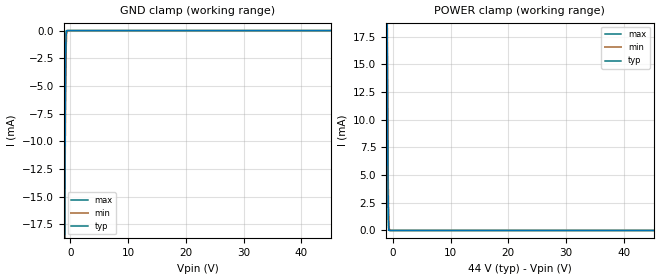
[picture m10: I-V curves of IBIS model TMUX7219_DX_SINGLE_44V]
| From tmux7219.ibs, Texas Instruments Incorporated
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[Model]   TMUX7219_DX_SINGLE_44V
Model_type   Terminator
|   typ   min   max
C_comp   45pF   45pF   45pF
[Voltage Range]   44   39.6   48.4
[Temperature Range]   27   125   -40
[Power Clamp Reference]   44   39.6   48.4
[GND Clamp Reference]   0   0   0
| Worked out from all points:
|   GND clamp passes 1 mA (typ) near -0.77 V on its own axis
|   POWER clamp passes 1 mA (typ) near -0.77 V on its own axis
[GND Clamp]
|   Voltage   I(typ)   I(min)   I(max)
-30V      -4.646A    -4.808A    -4.649A
-1.02V    -22.01mA   -24.41mA   -19.81mA
-930mV    -11.04mA   -13.89mA   -8.565mA
-840mV    -3.269mA   -5.934mA   -1.414mA
-750mV    -384.6uA   -1.761mA   -36.1uA
-660mV    -13.98uA   -270.8uA   -471.5nA
-570mV    -402.9nA   -19.98uA   -235.8nA
-210mV    0A         0A         0A
60V       0A         0A         0A
[POWER Clamp]
|   Voltage   I(typ)   I(min)   I(max)
-30V      4.646A     4.808A     4.649A
-1.02V    22.01mA    24.41mA    19.81mA
-930mV    11.04mA    13.89mA    8.565mA
-840mV    3.269mA    5.934mA    1.414mA
-750mV    384.6uA    1.761mA    36.1uA
-660mV    13.98uA    270.8uA    471.5nA
-570mV    402.9nA    19.98uA    235.8nA
-210mV    0A         0A         0A
60V       0A         0A         0A
